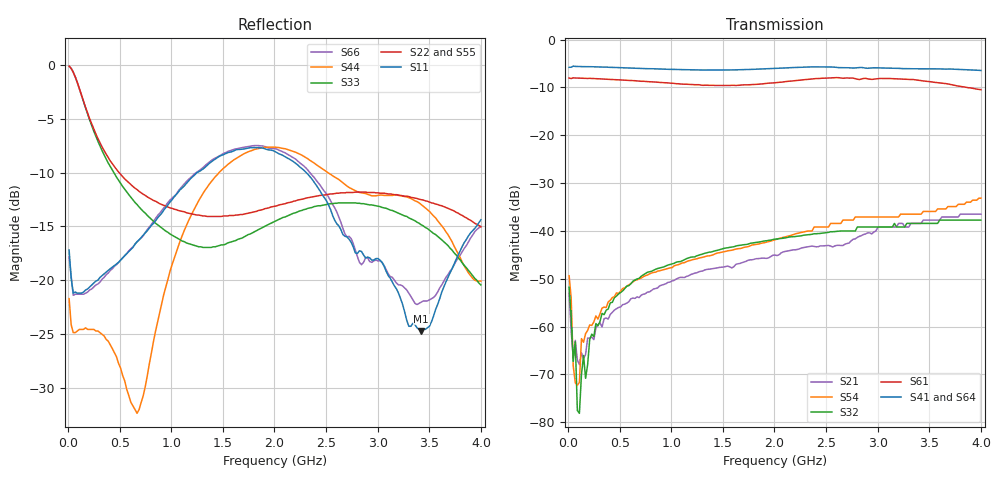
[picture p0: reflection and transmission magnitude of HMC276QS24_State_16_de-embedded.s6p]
! Hittite Microwave Corporation
! 20 Alpha Road
! Chelmsford, MA 01824
! Tel: 978-250-3343
! Fax: 978-250-3373
! Device: HMC276QS24, 0.7-3.0 GHz, GaAS MMIC 4x2 Switch Matrix in 24-lead QSOP package
! Misc: Data was de-embedded to package pins.
!  Port 1 = OP1
!  Port 2 = VL
!  Port 3 = VH
!  Port 4 = HH
!  Port 5 = HL
!  Port 6 = OP2
!  Vdd = +5 V
!  Vctl = 0 V[Logic 0] / +5 V[Logic 1]
!  State 16,  HH to OP1, HH to OP2
!  Control Lines (Logic)
!  HV 1 = 1, Tone 1 = 1
!  HV 2 = 1, Tone 2 = 1
!  Data reformated to new Touchstone file format - Wed Jan 10 16:02:56  2007
# MHz S DB R 50
! 6 Port Network Data
! freq  dbS11  angS11  dbS12  angS12  dbS13  angS13  dbS14  angS14
!  dbS15  angS15  dbS16  angS16
!  dbS21  angS21  dbS22  angS22
!  dbS23  angS23  dbS24  angS24  dbS25  angS25  dbS26  angS26
!  dbS31  angS31  dbS32  angS32  dbS33  angS33  dbS34  angS34
!  dbS35  angS35  dbS36  angS36
!  dbS41  angS41  dbS42  angS42
!  dbS43  angS43  dbS44  angS44  dbS45  angS45  dbS46  angS46
!  dbS51  angS51  dbS52  angS52  dbS53  angS53  dbS54  angS54
!  dbS55  angS55  dbS56  angS56
!  dbS61  angS61  dbS62  angS62
!  dbS63  angS63  dbS64  angS64  dbS65  angS65  dbS66  angS66
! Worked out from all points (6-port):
!   201 points, 10 MHz to 4 GHz, reference 50 ohm
!   strongest paths, dB at 10 MHz, 1.008 GHz, 2.005 GHz, 3.002 GHz, 4 GHz:
!     S41: -5.8, -6.2, -6.0, -5.9, -6.4
!     S64: -5.9, -6.2, -6.1, -5.9, -6.5
!     S61: -8.0, -9.1, -9.0, -8.2, -10.5
!     S32: -51.8, -46.9, -41.7, -39.2, -37.7
!     S54: -49.4, -47.7, -41.8, -37.1, -33.2
!     S21: -53.0, -50.5, -45.0, -39.2, -36.5
!   lowest |S11| = -24.7 dB at 3.421 GHz (marker M1), VSWR 1.12, Z = 54 + j4.54 ohm
!   |S11| at or under -10 dB: start of sweep to 1.248 GHz; 2.309 GHz to end of sweep
